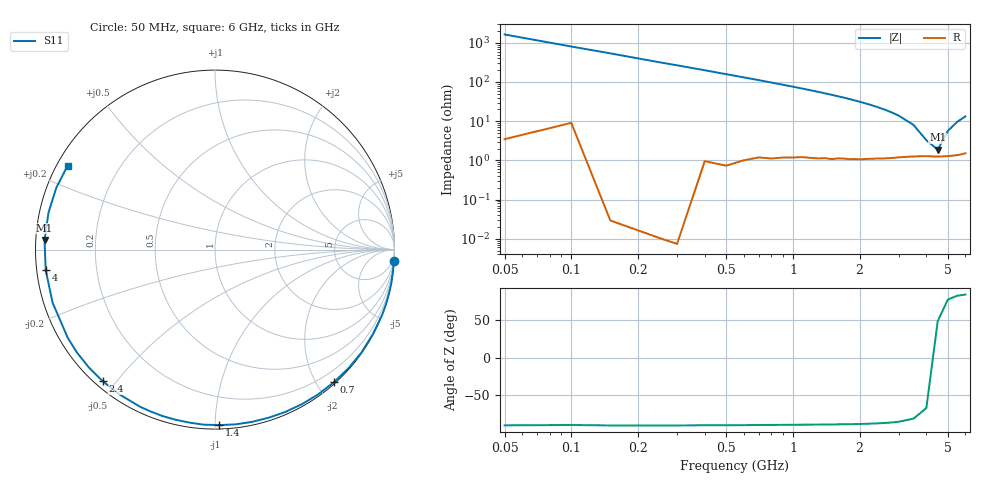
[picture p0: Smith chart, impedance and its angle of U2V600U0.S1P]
! SIEMENS Discrete & RF Semiconductors
! BBY52-02W
! Si Tuning Diode in SCD-80
! VR = 0.6 V
! S-Parameters:  September  1997
# GHz  S  MA  R  50
!  f  S11
! GHz  MAG  ANG
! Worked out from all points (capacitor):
!   34 points, 50 MHz to 6 GHz, reference 50 ohm
!   read as one part to ground: C = 1.97 pF near 50 MHz
!   lowest |Z| = 1.87 ohm at 4.5 GHz (marker M1)
!   series resonance near 4.342 GHz, so ESL is about 680 pH
!   S11 on the Smith chart (normalised r, x): 50 MHz: 0, -33; 700 MHz: 0.02, -2.24; 1.4 GHz: 0.02, -1.02; 2.4 GHz: 0.02, -0.46; 4 GHz: 0.03, -0.06; 6 GHz: 0.03, +0.26
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0.05  0.9999 -3.5
0.15  1 -10.6
0.3  1 -21.2
0.4  0.9978 -28.1
0.5  0.9973 -35.0
0.6  0.9949 -41.6
0.7  0.9921 -48.1
0.8  0.9906 -54.6
0.9  0.988 -60.7
1  0.9858 -66.6
1.1  0.9832 -72.4
1.2  0.9818 -78.0
1.3  0.9803 -83.4
1.4  0.978 -88.6
1.6  0.9745 -98.3
1.8  0.9724 -107.4
2  0.9699 -115.6
2.2  0.9666 -123.4
2.4  0.9639 -130.5
2.6  0.9617 -137.1
2.8  0.9594 -143.3
3  0.9564 -149.0
3.5  0.952 -161.9
4  0.9501 -173.1
4.5  0.9513 176.8
5  0.9504 167.4
5.5  0.9489 158.6
6  0.9449 150.3
